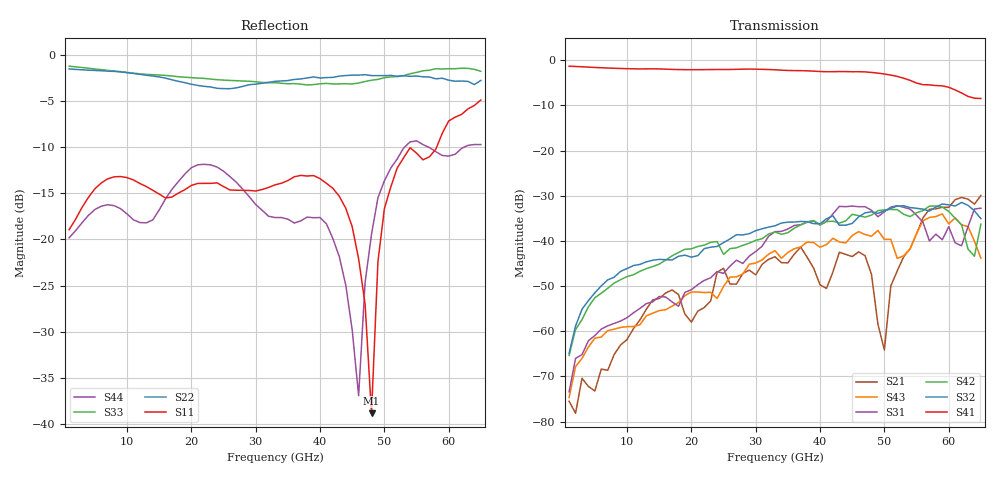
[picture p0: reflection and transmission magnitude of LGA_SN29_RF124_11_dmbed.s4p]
! Created Thu Nov 10 13:44:57 2022
# hz S ma R 50
! 4 Port Network Data from SP1.SP block
! freq  magS11  angS11  magS12  angS12  magS13  angS13  magS14  angS14
!  magS21  angS21  magS22  angS22  magS23  angS23  magS24  angS24
!  magS31  angS31  magS32  angS32  magS33  angS33  magS34  angS34
!  magS41  angS41  magS42  angS42  magS43  angS43  magS44  angS44
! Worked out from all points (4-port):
!   65 points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, 1 GHz to 65 GHz, reference 50 ohm
!   strongest paths, dB at 1 GHz, 17 GHz, 33 GHz, 49 GHz, 65 GHz:
!     S41: -1.3, -2.0, -2.1, -2.8, -8.5
!     S32: -64.9, -44.2, -36.6, -33.9, -35.1
!     S42: -65.3, -43.3, -38.0, -33.3, -36.3
!     S31: -73.4, -53.5, -37.9, -34.6, -32.7
!     S43: -74.7, -54.4, -42.2, -37.7, -43.8
!     S21: -75.5, -50.8, -43.5, -58.5, -29.9
!   lowest |S11| = -38.8 dB at 48 GHz (marker M1), VSWR 1.02, Z = 51 - j0.592 ohm
!   |S11| at or under -10 dB: start of sweep to 58.13 GHz
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1e9  0.1128 -30.2  4.091e-05 104.4  0.0001929 48.0  0.8628 -13.1
     0.000168 19.9  0.836 171.1  0.0006034 76.3  0.0005179 58.9
     0.0002134 52.6  0.0005708 65.7  0.8654 169.8  0.000246 85.9
     0.862 -13.1  0.0005408 70.3  0.000185 58.0  0.102 -29.6
1.4e10  0.1844 -176.4  0.002264 15.8  0.002228 -63.9  0.8059 -172.1
        0.002229 12.6  0.7658 54.5  0.00618 -33.3  0.005217 -80.1
        0.002117 -65.3  0.006118 -32.5  0.7781 43.9  0.001541 -65.0
        0.8053 -172.1  0.005208 -79.8  0.001585 -65.8  0.1274 -167.8
2.9e10  0.184 23.5  0.004654 156.3  0.006968 128.0  0.8022 2.7
        0.004755 161.7  0.6871 -113.4  0.01203 142.9  0.009105 90.1
        0.006787 126.6  0.01204 142.6  0.7174 -122.0  0.005329 119.4
        0.8008 2.6  0.009463 90.7  0.005529 119.5  0.1702 92.0
4.8e10  0.01146 -30.4  0.004496 142.5  0.02191 -122.7  0.7351 109.0
        0.004251 133.7  0.7695 63.8  0.02133 -54.5  0.01956 -126.8
        0.02187 -122.6  0.02108 -54.6  0.7268 26.1  0.01186 -114.2
        0.7347 108.9  0.01936 -127.4  0.01129 -112.7  0.1066 119.7
5e10  0.1465 -99.3  0.0002309 -0.3  0.02096 -128.7  0.7062 79.5
      0.0006181 -156.5  0.7689 47.9  0.02134 -69.5  0.0216 -150.9
      0.02109 -129.2  0.02155 -68.7  0.7495 3.8  0.01073 -154.2
      0.7056 79.4  0.02211 -152.2  0.0104 -154.5  0.2073 82.6
5.1e10  0.1924 -119.0  0.004165 -178.3  0.02401 -147.1  0.6872 64.6
        0.00318 -171.8  0.7716 39.5  0.02342 -82.6  0.0231 -168.3
        0.0237 -145.1  0.02302 -82.9  0.7575 -8.5  0.009878 -175.7
        0.6863 64.4  0.0223 -167.7  0.01042 -174.6  0.2432 69.3
6.5e10  0.5679 146.1  0.03315 -104.7  0.02172 156.9  0.3782 -127.0
        0.03189 -102.8  0.7248 -131.4  0.01719 95.8  0.01554 67.4
        0.02305 156.5  0.01764 97.0  0.8117 -140.3  0.006647 -66.9
        0.3777 -127.1  0.01531 71.2  0.00644 -67.8  0.326 149.8
